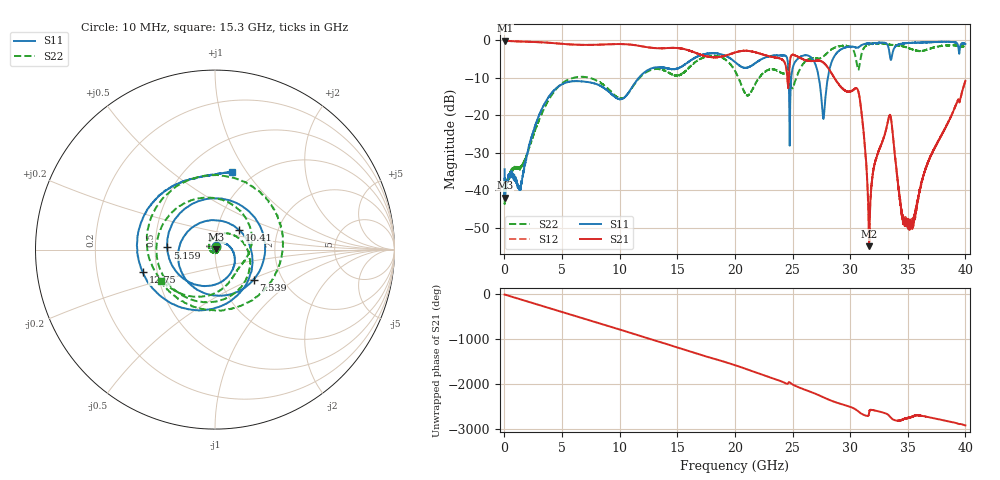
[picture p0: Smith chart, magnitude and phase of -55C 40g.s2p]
!Keysight Technologies,N5234A,MY52241180,A.10.60.03
!Date: Tuesday, February 27, 2024 08:55:02
!Correction: S11(Full 2 Port(1,2))
!S21(Full 2 Port(1,2))
!S12(Full 2 Port(1,2))
!S22(Full 2 Port(1,2))
!S2P File: Measurements: S11, S21, S12, S22:
# Hz S  dB  R 50
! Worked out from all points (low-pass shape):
!   6401 points, 10 MHz to 40 GHz, reference 50 ohm
!   highest |S21| = -0.04 dB at 16.25 MHz (marker M1); lowest = -54.9 dB at 31.65 GHz (marker M2)
!   |S21| within 3 dB of the highest: start of sweep to 16.34 GHz; 20.22 GHz to 21.55 GHz (1.326 GHz wide, 6.35 % of centre)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
!   lowest |S11| = -41.9 dB at 53.74 MHz (marker M3), VSWR 1.02, Z = 50.8 + j0.133 ohm
!   |S11| at or under -10 dB: start of sweep to 11.66 GHz; 24.66 GHz to 24.89 GHz (221.2 MHz wide, 0.893 % of centre); 27.28 GHz to 28.06 GHz (773.5 MHz wide, 2.8 % of centre)
!   |S22| runs from -43.6 to -0.7 dB; largest |S21 - S12| = 0.0086
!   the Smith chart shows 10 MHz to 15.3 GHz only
!   S11 on the Smith chart (normalised r, x): 10 MHz: 1.01, +0.04; 5.159 GHz: 0.58, +0.01; 7.539 GHz: 1.44, -0.52; 10.41 GHz: 1.27, +0.29; 12.75 GHz: 0.41, -0.13; 15.3 GHz: 0.80, +0.86
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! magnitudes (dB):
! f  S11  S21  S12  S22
! 10 MHz  -34.4  -0.1  0.0  -37.8
! 16.25 MHz  -41.3  0.0  0.0  -43.6
! 53.74 MHz  -41.9  -0.1  -0.1  -40.8
! 1.341 GHz  -39.5  -0.3  -0.3  -33.9
! 5.159 GHz  -11.5  -1.0  -1.0  -11.1
! 6.677 GHz  -10.9  -1.2  -1.2  -9.7
! 7.539 GHz  -11.3  -1.2  -1.2  -10.2
! 10.41 GHz  -15.2  -1.0  -1.0  -15.1
! 12.75 GHz  -7.5  -2.0  -2.0  -7.9
! 13.34 GHz  -7.2  -2.1  -2.1  -7.6
! 15.3 GHz  -7.1  -2.1  -2.2  -9.2
! 20 GHz  -5.8  -3.2  -3.2  -8.2
! 24.83 GHz  -13.2  -4.6  -4.5  -11.4
! 26.67 GHz  -4.7  -5.5  -5.5  -4.8
! 27.68 GHz  -20.9  -5.9  -5.9  -4.3
! 28.62 GHz  -4.3  -10.0  -9.9  -2.0
! 30.65 GHz  -1.9  -13.1  -13.2  -7.5
! 31.65 GHz  -0.8  -54.9  -53.8  -1.1
! 33.34 GHz  -2.1  -20.7  -20.7  -1.0
! 34.55 GHz  -0.8  -47.1  -46.5  -1.6
! 35.28 GHz  -0.7  -50.2  -49.0  -2.3
! 40 GHz  -1.0  -10.8  -10.8  -1.8
